FUNCTION_BLOCK FB_GetPagedProducts

VAR_IN_OUT
	fbClient:FB_IotHttpClient;
END_VAR
VAR_OUTPUT
	bBusy:BOOL;
	bError:BOOL;
	
END_VAR
VAR
	fbRequest			: FB_IotHttpRequest;
	fbJson				: FB_JsonDomParser;
	nState				: UDINT;
	SearchRisingEdge			: R_TRIG;
	NextPageRisingEdge			: R_TRIG;
	PreviousPageRisingEdge			: R_TRIG;
	emptyProducts:ARRAY[1..PageSize] OF ST_Product;
	
	sUri:STRING;
	
	fbJsonDomParser		:FB_JsonDomParser;
	jsonDoc			:SJsonValue;
	productArrayJsonDoc:SJsonValue;
	index:INT;
	arraySize:UDINT;
	productJsonDoc:SJsonValue;
	//HMI
	bSearch:BOOL;
	bNextPage:BOOL;
	bPreviousPage:BOOL;
	
	nCurrentPage:DINT;
	nTotalItems:DINT;
	nTotalPages:DINT;
	
	products:ARRAY[1..PageSize] OF ST_Product;
END_VAR
VAR CONSTANT
	PageSize:INT:=10;
END_VAR

SearchRisingEdge(CLK:=bSearch , Q=> );
NextPageRisingEdge(CLK:=bNextPage , Q=> );
PreviousPageRisingEdge(CLK:=bPreviousPage , Q=> );
CASE nState OF
	0:
		IF SearchRisingEdge.Q THEN
			nCurrentPage:=1;
			nState:= 5;
		END_IF
		IF NextPageRisingEdge.Q AND nCurrentPage<nTotalPages THEN
			nCurrentPage:=nCurrentPage+1;
			nState:= 5;
		END_IF
		IF PreviousPageRisingEdge.Q AND nCurrentPage>1 THEN
			nCurrentPage:=nCurrentPage-1;
			nState:= 5;
		END_IF
	5:	
		products:=emptyProducts;
		sUri:=CONCAT('/Product/paged?pageNumber=',DINT_TO_STRING(nCurrentPage));
		sUri:=CONCAT(sUri,'&pageSize=10');
		
		IF fbRequest.SendRequest(sUri:=sUri, fbClient:=fbClient, eRequestType:=ETcIotHttpRequestType.HTTP_Get, 0, 0, 0) THEN				
				nState:= 10;
				bBusy:= TRUE;
				bError:= FALSE;
				
		END_IF
	10:
		IF NOT fbRequest.bBusy THEN
			bError:=TRUE;
			IF NOT fbRequest.bError THEN
				bError:=FALSE;
				
				IF fbRequest.nStatusCode=200 THEN
					jsonDoc:=fbRequest.GetJsonDomContent(fbJsonDomParser);
					IF jsonDoc<>0 THEN
						nTotalItems:=fbJsonDomParser.GetInt(fbJsonDomParser.FindMember(jsonDoc,'totalItems'));
						nTotalPages:=fbJsonDomParser.GetInt(fbJsonDomParser.FindMember(jsonDoc,'totalPages'));
						productArrayJsonDoc:=fbJsonDomParser.FindMember(jsonDoc,'items');
						arraySize:=fbJsonDomParser.GetArraySize(productArrayJsonDoc);
						FOR index:=0 TO UDINT_TO_INT(arraySize) DO
							productJsonDoc:=fbJsonDomParser.GetArrayValueByIdx(idx:=index,v:=productArrayJsonDoc);
							products[index+1].Id:=fbJsonDomParser.GetInt(fbJsonDomParser.FindMember(productJsonDoc,'id'));
							products[index+1].CreatDateTime:=fbJsonDomParser.GetDateTime(fbJsonDomParser.FindMember(productJsonDoc,'creatDateTime'));
							products[index+1].BarCode:=fbJsonDomParser.GetString(fbJsonDomParser.FindMember(productJsonDoc,'barCode'));
							products[index+1].FinalPressure:=fbJsonDomParser.GetDouble(fbJsonDomParser.FindMember(productJsonDoc,'finalPressure'));
							products[index+1].FinalDisplacement:=fbJsonDomParser.GetDouble(fbJsonDomParser.FindMember(productJsonDoc,'finalDisplacement'));
							products[index+1].IsQualified:=fbJsonDomParser.GetBool(fbJsonDomParser.FindMember(productJsonDoc,'isQualified'));
						END_FOR
						nState:=100;
					END_IF
				END_IF
			END_IF
		END_IF
	100:
		nState:=0;
END_CASE

END_FUNCTION_BLOCK
